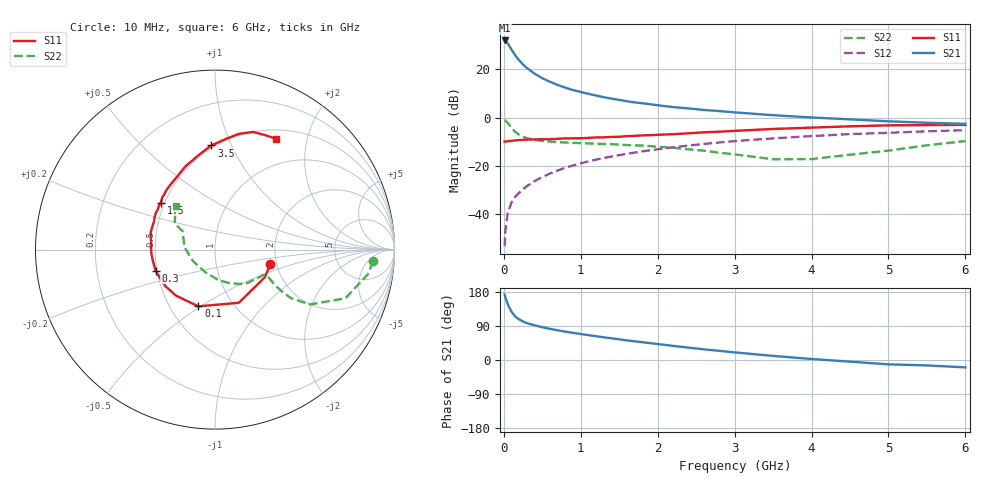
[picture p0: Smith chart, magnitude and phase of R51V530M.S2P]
! SIEMENS Small Signal Semiconductors
! BFR183
! Si NPN RF Bipolar Junction Transistor in SOT23
! VCE = 1.5 V  IC = 30 mA
! Common Emitter S-Parameters:  May  1996
# GHz  S  MA  R  50
!  f  S11  S21  S12  S22
! GHz  MAG  ANG  MAG  ANG  MAG  ANG  MAG  ANG
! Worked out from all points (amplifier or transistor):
!   36 points, 10 MHz to 6 GHz, reference 50 ohm
!   highest |S21| = 31.9 dB at 10 MHz (marker M1)
!   |S21| within 3 dB of that: start of sweep to 84.95 MHz
!   unconditionally stable (mu >= 1): start of sweep to 11.91 MHz; 296 MHz to 2.713 GHz
!   at 250 MHz: K = 0.96, MSG = 25.7 dB, |S12| = -29.6 dB
!   at 1.4 GHz: K = 1.10, MAG = 10.1 dB, |S12| = -16.1 dB
!   at 6 GHz: K = 0.96, MSG = 1.3 dB, |S12| = -5.2 dB
!   S11 on the Smith chart (normalised r, x): 10 MHz: 1.85, -0.34; 100 MHz: 0.69, -0.49; 300 MHz: 0.49, -0.13; 1.5 GHz: 0.48, +0.30; 3.5 GHz: 0.48, +0.84; 6 GHz: 0.62, +1.51
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0.01  0.3192 -15.0  39.14 172.8  0.0022 83.9  0.8832 -4.3
0.02  0.3171 -29.2  38.46 165.6  0.0047 78.6  0.8633 -9.1
0.05  0.3247 -65.8  34.04 147.5  0.0106 74.6  0.7752 -20.5
0.1  0.3294 -106.3  25.36 127.2  0.0175 68.6  0.6111 -30.0
0.15  0.3365 -130.4  19.11 114.6  0.0233 66.6  0.5027 -32.6
0.2  0.3433 -143.6  15.19 107.1  0.028 68.5  0.4404 -32.1
0.25  0.3453 -153.3  12.45 101.6  0.0333 69.5  0.4008 -31.0
0.3  0.3508 -160.6  10.54 97.4  0.0383 70.5  0.3756 -30.0
0.4  0.3529 -171.6  8.071 91.6  0.0487 71.9  0.3445 -28.0
0.5  0.3559 -178.1  6.514 86.5  0.0589 72.3  0.3271 -27.0
0.6  0.357 174.9  5.478 82.2  0.0698 72.3  0.3185 -26.8
0.7  0.3636 169.9  4.717 78.3  0.0807 72.5  0.311 -27.3
0.8  0.371 164.8  4.137 74.8  0.0918 71.7  0.3044 -27.8
0.9  0.3717 160.8  3.704 71.7  0.1025 71.0  0.299 -28.5
1.1  0.3798 152.8  3.09 65.7  0.1244 69.2  0.2926 -31.5
1.5  0.3995 139.0  2.315 54.6  0.1675 65.1  0.2768 -38.0
2.2  0.4527 119.0  1.647 37.3  0.2428 56.7  0.2375 -53.8
2.6  0.4952 108.9  1.433 28.2  0.2847 51.3  0.2065 -65.7
3.5  0.5809 92.0  1.119 10.8  0.3709 38.3  0.1374 -113.2
4.5  0.6587 78.3  0.916 -4.4  0.4553 24.6  0.1706 175.4
5.5  0.697 65.9  0.779 -14.3  0.5195 12.3  0.2665 147.2
6  0.7046 61.1  0.742 -19.5  0.5475 4.7  0.3273 132.2
